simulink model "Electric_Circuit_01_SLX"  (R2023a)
settings: Solver=ode23s  StartTime=0.0  StopTime=10.0  MaxStep=0.001  RelTol=1e-3
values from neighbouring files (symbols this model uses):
  C_2 = 0.001*F    (= 0.001)    [Electric_Circuit_01_EQN.m]    (also in Electric_Circuit_01_SLX_m.m; Electric_Circuit_04_EQN.m; Electric_Circuit_04_SLX_m.m; Electric_Circuit_05_EQN.m)
  C_4 = 0.001*F    (= 0.001)    [Electric_Circuit_01_EQN.m]    (also in Electric_Circuit_01_SLX_m.m; Electric_Circuit_06_EQN.m; Electric_Circuit_06_SLX_m.m; Electric_Circuit_09_EQN.m)
  C_6 = 0.001*F    (= 0.001)    [Electric_Circuit_01_EQN.m]    (also in Electric_Circuit_01_SLX_m.m; Electric_Circuit_03_EQN.m; Electric_Circuit_03_SLX_m.m; Electric_Circuit_06_EQN.m)
  I_1_0 = 10*A    (= 10)    [Electric_Circuit_01_SLX_m.m]
  I_5_0 = 0*A    (= 0)    [Electric_Circuit_01_SLX_m.m]    (also in BIG_EC_Simscape_SLX_m.m; Electric_Circuit_06_SLX_m.m; Electric_Circuit_09_SLX_m.m; Electric_Circuit_10_SLX_m.m)
  I_7_0 = 0*A    (= 0)    [Electric_Circuit_01_SLX_m.m]    (also in Electric_Circuit_09_SLX_m.m; Inductive_Circuit_2_SLX_m.m)
  L_5 = 0.002*H    (= 0.002)    [Electric_Circuit_01_EQN.m]    (also in Electric_Circuit_01_SLX_m.m; BIG_EC_Simscape_EQN.m; BIG_EC_Simscape_SLX_m.m; Electric_Circuit_06_EQN.m)
  R_3 = 100*Ohm    (= 100)    [Electric_Circuit_01_EQN.m]    (also in Electric_Circuit_01_SLX_m.m; Electric_Circuit_02_EQN.m; Electric_Circuit_02_SLX_m.m; Electric_Circuit_04_EQN.m)
  Ts = Tfin/Nr_Ts_Points    (= 0.005)    [Electric_Circuit_01_SLX_m.m]    (also in BIG_EC_Simscape_SLX_m.m = 0.0003; Car_Dumper_SLX_m.m = 0.0022779; Electric_Circuit_02_SLX_m.m = 0.000480145; Electric_Circuit_03_SLX_m.m = 0.0006)
  V_2_0 = 0*V    (= 0)    [Electric_Circuit_01_SLX_m.m]    (also in Electric_Circuit_04_SLX_m.m; Electric_Circuit_05_SLX_m.m)
  V_4_0 = 0*V    (= 0)    [Electric_Circuit_01_SLX_m.m]    (also in Electric_Circuit_06_SLX_m.m; Electric_Circuit_09_SLX_m.m)
  V_6_0 = 0*V    (= 0)    [Electric_Circuit_01_SLX_m.m]    (also in Electric_Circuit_03_SLX_m.m; Electric_Circuit_06_SLX_m.m; Electric_Circuit_08_SLX_m.m; Electric_Circuit_10_SLX_m.m)

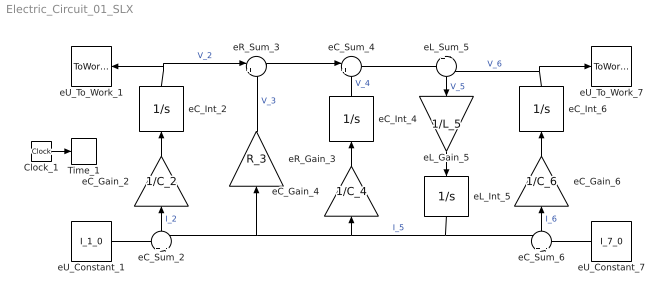
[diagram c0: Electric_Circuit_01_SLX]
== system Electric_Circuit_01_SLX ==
  Clock_1 : Clock
  Time_1 : ToWorkspace  VariableName=t  SaveFormat=Timeseries  SampleTime=Ts
  eC_Gain_2 : Gain  Gain=1/C_2  Multiplication=Matrix(K*u)
  eC_Gain_4 : Gain  Gain=1/C_4  Multiplication=Matrix(K*u)
  eC_Gain_6 : Gain  Gain=1/C_6  Multiplication=Matrix(K*u)
  eC_Int_2 : Integrator  InitialCondition=V_2_0
  eC_Int_4 : Integrator  InitialCondition=V_4_0
  eC_Int_6 : Integrator  InitialCondition=V_6_0
  eC_Sum_2 : Sum  Inputs=+|-
  eC_Sum_4 : Sum  Inputs=|+-
  eC_Sum_6 : Sum  Inputs=+|-
  eL_Gain_5 : Gain  Gain=1/L_5  Multiplication=Matrix(K*u)
  eL_Int_5 : Integrator  InitialCondition=I_5_0
  eL_Sum_5 : Sum  Inputs=+|-
  eR_Gain_3 : Gain  Gain=R_3  Multiplication=Matrix(K*u)
  eR_Sum_3 : Sum  Inputs=|+-
  eU_Constant_1 : Constant  Value=I_1_0
  eU_Constant_7 : Constant  Value=I_7_0
  eU_To_Work_1 : ToWorkspace  VariableName=V_1_0  SaveFormat=Timeseries  SampleTime=Ts
  eU_To_Work_7 : ToWorkspace  VariableName=V_7_0  SaveFormat=Timeseries  SampleTime=Ts
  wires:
  eU_Constant_1/1 -> eC_Sum_2/1
  eL_Int_5/1 -> eC_Sum_2/2, eR_Gain_3/1, eC_Gain_4/1, eC_Sum_6/1  "I_5"
  eC_Int_2/1 -> eU_To_Work_1/1, eR_Sum_3/1  "V_2"
  eC_Sum_2/1 -> eC_Gain_2/1  "I_2"
  eC_Gain_2/1 -> eC_Int_2/1
  eR_Sum_3/1 -> eC_Sum_4/1
  eR_Gain_3/1 -> eR_Sum_3/2  "V_3"
  eC_Sum_4/1 -> eL_Sum_5/1
  eC_Gain_4/1 -> eC_Int_4/1
  eC_Int_4/1 -> eC_Sum_4/2  "V_4"
  eC_Int_6/1 -> eL_Sum_5/2, eU_To_Work_7/1  "V_6"
  eL_Sum_5/1 -> eL_Gain_5/1  "V_5"
  eL_Gain_5/1 -> eL_Int_5/1
  eU_Constant_7/1 -> eC_Sum_6/2
  eC_Sum_6/1 -> eC_Gain_6/1  "I_6"
  eC_Gain_6/1 -> eC_Int_6/1
  Clock_1/1 -> Time_1/1
